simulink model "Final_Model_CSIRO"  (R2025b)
settings: Solver=ode23tb  StartTime=0.0  StopTime=50  RelTol=1e-3
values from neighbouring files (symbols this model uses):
  C_4 = 0.1670*C_b    (= 1.00487241952e-06)    [VSM_CSIRO.m]    (also in VSM.m)
  C_6 = 0.2835*C_b    (= 1.70587623314e-06)    [VSM_CSIRO.m]    (also in VSM.m)
  C_8 = 0.2275*C_b    (= 1.36891302659e-06)    [VSM_CSIRO.m]    (also in VSM.m)
  C_dc = 0.008*(n)    (= 1.6)    [VSM_CSIRO.m]    (also in VSM.m)
  C_f = n*300*10^-6    (= 0.06)    [VSM_CSIRO.m]    (also in VSM.m)
  D_p = (1/(m_p*w_b))    (= 101321.183642)    [VSM_CSIRO.m]    (also in VSM.m)
  droop_percentage = 1    [VSM_CSIRO.m]    (also in VSM.m = 5)
  i_ll = -1.15*(S_b/Vdc_n)-i_loss_dc    [VSM_CSIRO.m]    (also in VSM.m)
  i_ul = 1.15*(S_b/Vdc_n)+i_loss_dc    [VSM_CSIRO.m]    (also in VSM.m)
  J = D_p*tau_f    (= 2026.42367285)    [VSM_CSIRO.m]    (also in VSM.m)
  k_dc = eta_1/(Vdc_n*m_p)    [VSM_CSIRO.m]    (also in VSM.m)
  K_p = (1/Vdc_n)    [VSM_CSIRO.m]    (also in VSM.m)
  K_r = 1/R_dc    [VSM_CSIRO.m]    (also in VSM.m)
  Kff_i = 1    [VSM_CSIRO.m]    (also in VSM.m)
  Kff_v = 1    [VSM_CSIRO.m]    (also in VSM.m)
  Ki_i = (1/n)*1.19    (= 0.00595)    [VSM_CSIRO.m]    (also in VSM.m)
  Ki_v = (n)*1.161022    (= 232.2044)    [VSM_CSIRO.m]    (also in VSM.m)
  ki_v_ac = 4*5.2500e-04    (= 0.0021)    [VSM_CSIRO.m]    (also in VSM.m)
  Kp_i = 0.738891    [VSM_CSIRO.m]    (also in VSM.m)
  Kp_v = 0.52    [VSM_CSIRO.m]    (also in VSM.m)
  kp_v_ac = 0.001    [VSM_CSIRO.m]    (also in VSM.m)
  L1_pu = 1*0.0186/m    (= 0.000186)    [VSM_CSIRO.m]    (also in VSM.m)
  L_45 = L_lines(2)    [VSM_CSIRO.m]    (also in VSM.m)
  L_56 = L_lines(3)    [VSM_CSIRO.m]    (also in VSM.m)
  L_67 = L_lines(5)    [VSM_CSIRO.m]    (also in VSM.m)
  L_78 = L_lines(6)    [VSM_CSIRO.m]    (also in VSM.m)
  L_89 = L_lines(8)    [VSM_CSIRO.m]    (also in VSM.m)
  L_94 = L_lines(9)    [VSM_CSIRO.m]    (also in VSM.m)
  L_f = (1/n)*200*10^-6    (= 1e-06)    [VSM_CSIRO.m]    (also in VSM.m)
  n = 200    [VSM_CSIRO.m]    (also in VSM.m)
  pl = S_b*ps    (= 75000000)    [VSM_CSIRO.m]    (also in VSM.m)
  ps = base/3    (= 0.75)    [VSM_CSIRO.m]    (also in VSM.m)
  R1_pu = 1*0.00734/m    (= 7.34e-05)    [VSM_CSIRO.m]    (also in VSM.m)
  R_45 = R_lines(2)    [VSM_CSIRO.m]    (also in VSM.m)
  R_56 = R_lines(3)    [VSM_CSIRO.m]    (also in VSM.m)
  R_67 = R_lines(5)    [VSM_CSIRO.m]    (also in VSM.m)
  R_78 = R_lines(6)    [VSM_CSIRO.m]    (also in VSM.m)
  R_89 = R_lines(8)    [VSM_CSIRO.m]    (also in VSM.m)
  R_94 = R_lines(9)    [VSM_CSIRO.m]    (also in VSM.m)
  R_dc = (Vdc_n/(0.05*(S_b)/Vdc_n))    [VSM_CSIRO.m]    (also in VSM.m)
  R_f = 0.001/n    (= 5e-06)    [VSM_CSIRO.m]    (also in VSM.m)
  S_b = 100*(10^6)    (= 100000000)    [VSM_CSIRO.m]    (also in VSM.m)
  S_bt = S_b    (= 100000000)    [VSM_CSIRO.m]    (also in VSM.m)
  T_en = T_load-0.5    (= 44.5)    [VSM_CSIRO.m]    (also in VSM.m = 24.5)
  t_l = 2    [VSM_CSIRO.m]
  tau_dc = 0.05    [VSM_CSIRO.m]    (also in VSM.m)
  tau_g = 5    [VSM_CSIRO.m]    (also in VSM.m)
  V1_rms = 1000    [VSM_CSIRO.m]    (also in VSM.m)
  V2_rms = 13800    [VSM_CSIRO.m]    (also in VSM.m)
  V_m = sqrt(2/3)*V1_rms    [VSM_CSIRO.m]    (also in VSM.m)
  Vdc_n = 3*V_m    [VSM_CSIRO.m]    (also in VSM.m)
  w_b = 2*pi*f_b    (= 314.159265359)    [VSM_CSIRO.m]    (also in VSM.m)
  w_f = 2*pi*5    (= 31.4159265359)    [VSM_CSIRO.m]    (also in VSM.m)
undefined symbols (not defined in the file or in its folder): D1, Delta, DiscIntNeverNeededParam, i_dc
libraries: spsSeriesRLCBranchLib x142, spsThreePhaseVIMeasurementLib x69, slpidlib x44, spsabctodq0Lib x44, spsVoltageMeasurementLib x28, spsGroundLib x23, spsThreePhaseBreakerLib x23, spsThreePhaseParallelRLCLoadLib x21, spsdq0toabcLib x16, spsUniversalBridgeLib x16, spsPowerPositiveSequenceLib x14, spsDCVoltageSourceLib x14
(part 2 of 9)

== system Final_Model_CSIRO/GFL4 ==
  B1 : spsThreePhaseVIMeasurementLib/Three-Phase V-I Measurement  VoltageMeasurement=phase-to-ground  SetLabelV=on  LabelV=Vabc_B1_5  Vpu=off  VpuLL=off  CurrentMeasurement=yes  SetLabelI=on  LabelI=Iabc_B1_5  Ipu=off  Pbase=100e6  Vbase=500e3  OutputType=Complex  PhasorSimulation=off  PSBequivalent=0
  B3 : spsThreePhaseVIMeasurementLib/Three-Phase V-I Measurement  VoltageMeasurement=phase-to-ground  SetLabelV=on  LabelV=Vabc_B3_5  Vpu=off  VpuLL=off  CurrentMeasurement=yes  SetLabelI=on  LabelI=Iabc_B3_5  Ipu=off  Pbase=100e6  Vbase=500e3  OutputType=Complex  PhasorSimulation=off  PSBequivalent=0
  B4 : spsThreePhaseVIMeasurementLib/Three-Phase V-I Measurement  VoltageMeasurement=phase-to-ground  SetLabelV=on  LabelV=Vabc_B4_5  Vpu=off  VpuLL=off  CurrentMeasurement=yes  SetLabelI=on  LabelI=Iabc_B4_5  Ipu=off  Pbase=100e6  Vbase=500e3  OutputType=Complex  PhasorSimulation=off  PSBequivalent=0
  Constant1 : Constant  Value=0  SampleTime=-1
  Gain2 : Gain  Gain=1e-8
  Inverter Control : Subsystem
  LCL Filter : Subsystem
  Power (Positive-Sequence) : spsPowerPositiveSequenceLib/Power (Positive-Sequence)  Freq=50  Vinit=[0, 0]  Iinit=[0, 0]  Ts=0
  Scope : Scope  NumInputPorts=4
  Scope1 : Scope
  Step : Step  Time=12+3*t_l  After=8200  SampleTime=0
  Universal Bridge : spsUniversalBridgeLib/Universal Bridge  Arms=3  SnubberResistance=1e5  SnubberCapacitance=inf  Device=Average-model based VSC  Ron=1e-3  Lon=0  ForwardVoltages="[  0  0  ]"  ForwardVoltage=0  GTOparameters=[ 10e-6 , 20e-6 ]  IGBTparameters=[ 1e-6 , 2e-6 ]  Measurements=None  Measurements_2=None  converterType=Rectifier
  Vdc : spsDCVoltageSourceLib/DC Voltage Source  Amplitude=1800  Measurements=None
  Voltage Measurement1 : spsVoltageMeasurementLib/Voltage Measurement  PhasorSimulation=off  OutputType=Complex  PSBequivalent=0
  Connection Port : PMIOPort  Side=Left
  Connection Port1 : PMIOPort  Port=2  Side=Left
  Connection Port2 : PMIOPort  Port=3  Side=Left
  Out1 : Outport
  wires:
  [Vabc_B1_5] -> Scope/3  "Inverter Voltage"
  [Iabc_B1_5] -> Scope/4  "Inverter Current"
  Voltage Measurement1/1 -> Scope1/1
  [Iabc_B3_5] -> Power (Positive-Sequence)/2, Scope/2  "PCC Current"
  Inverter Control/1(Pulses) -> Universal Bridge/1
  [Vabc_B3_5] -> Inverter Control/1(Vabc_B3)
  [Iabc_B3_5] -> Inverter Control/2(Iabc_B3)
  [Vabc_B3_5] -> Scope/1, Power (Positive-Sequence)/1  "PCC Voltage"
  Power (Positive-Sequence)/1 -> Gain2/1
  Gain2/1 -> Out1/1
  Constant1/1 -> Inverter Control/4(Iqref)
  Step/1 -> Inverter Control/3(Idref)
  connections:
  Universal Bridge/RConn1 -- Vdc/RConn1
  Universal Bridge/RConn2 -- Vdc/LConn1
  B1/LConn2 -- Voltage Measurement1/LConn2 -- Universal Bridge/LConn2
  Universal Bridge/LConn1 -- Voltage Measurement1/LConn1 -- B1/LConn1
  B3/LConn3 -- LCL Filter/RConn3
  B3/RConn3 -- B4/LConn3
  B3/RConn1 -- B4/LConn1
  Connection Port2/RConn1 -- B4/RConn3
  B3/LConn2 -- LCL Filter/RConn2
  Universal Bridge/LConn3 -- B1/LConn3
  B3/RConn2 -- B4/LConn2
  B3/LConn1 -- LCL Filter/RConn1
  B1/RConn1 -- LCL Filter/LConn1
  B1/RConn2 -- LCL Filter/LConn2
  B1/RConn3 -- LCL Filter/LConn3
  B4/RConn1 -- Connection Port/RConn1
  B4/RConn2 -- Connection Port1/RConn1

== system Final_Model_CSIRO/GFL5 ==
  B1 : spsThreePhaseVIMeasurementLib/Three-Phase V-I Measurement  VoltageMeasurement=phase-to-ground  SetLabelV=on  LabelV=Vabc_B1_6  Vpu=off  VpuLL=off  CurrentMeasurement=yes  SetLabelI=on  LabelI=Iabc_B1_6  Ipu=off  Pbase=100e6  Vbase=500e3  OutputType=Complex  PhasorSimulation=off  PSBequivalent=0
  B3 : spsThreePhaseVIMeasurementLib/Three-Phase V-I Measurement  VoltageMeasurement=phase-to-ground  SetLabelV=on  LabelV=Vabc_B3_6  Vpu=off  VpuLL=off  CurrentMeasurement=yes  SetLabelI=on  LabelI=Iabc_B3_6  Ipu=off  Pbase=100e6  Vbase=500e3  OutputType=Complex  PhasorSimulation=off  PSBequivalent=0
  B4 : spsThreePhaseVIMeasurementLib/Three-Phase V-I Measurement  VoltageMeasurement=phase-to-ground  SetLabelV=on  LabelV=Vabc_B4_6  Vpu=off  VpuLL=off  CurrentMeasurement=yes  SetLabelI=on  LabelI=Iabc_B4_6  Ipu=off  Pbase=100e6  Vbase=500e3  OutputType=Complex  PhasorSimulation=off  PSBequivalent=0
  Constant1 : Constant  Value=0  SampleTime=-1
  Gain2 : Gain  Gain=1e-8
  Inverter Control : Subsystem
  LCL Filter : Subsystem
  Power (Positive-Sequence) : spsPowerPositiveSequenceLib/Power (Positive-Sequence)  Freq=50  Vinit=[0, 0]  Iinit=[0, 0]  Ts=0
  Scope : Scope  NumInputPorts=4
  Scope1 : Scope
  Step : Step  Time=12+4*t_l  After=8200  SampleTime=0
  Universal Bridge : spsUniversalBridgeLib/Universal Bridge  Arms=3  SnubberResistance=1e5  SnubberCapacitance=inf  Device=Average-model based VSC  Ron=1e-3  Lon=0  ForwardVoltages="[  0  0  ]"  ForwardVoltage=0  GTOparameters=[ 10e-6 , 20e-6 ]  IGBTparameters=[ 1e-6 , 2e-6 ]  Measurements=None  Measurements_2=None  converterType=Rectifier
  Vdc : spsDCVoltageSourceLib/DC Voltage Source  Amplitude=1800  Measurements=None
  Voltage Measurement1 : spsVoltageMeasurementLib/Voltage Measurement  PhasorSimulation=off  OutputType=Complex  PSBequivalent=0
  Connection Port : PMIOPort  Side=Left
  Connection Port1 : PMIOPort  Port=2  Side=Left
  Connection Port2 : PMIOPort  Port=3  Side=Left
  Out1 : Outport
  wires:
  [Vabc_B1_6] -> Scope/3  "Inverter Voltage"
  [Iabc_B1_6] -> Scope/4  "Inverter Current"
  Voltage Measurement1/1 -> Scope1/1
  [Iabc_B3_6] -> Power (Positive-Sequence)/2, Scope/2  "PCC Current"
  Inverter Control/1(Pulses) -> Universal Bridge/1
  [Vabc_B3_6] -> Inverter Control/1(Vabc_B3)
  [Iabc_B3_6] -> Inverter Control/2(Iabc_B3)
  [Vabc_B3_6] -> Scope/1, Power (Positive-Sequence)/1  "PCC Voltage"
  Power (Positive-Sequence)/1 -> Gain2/1
  Gain2/1 -> Out1/1
  Constant1/1 -> Inverter Control/4(Iqref)
  Step/1 -> Inverter Control/3(Idref)
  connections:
  Universal Bridge/RConn1 -- Vdc/RConn1
  Universal Bridge/RConn2 -- Vdc/LConn1
  B1/LConn2 -- Voltage Measurement1/LConn2 -- Universal Bridge/LConn2
  Universal Bridge/LConn1 -- Voltage Measurement1/LConn1 -- B1/LConn1
  B3/LConn3 -- LCL Filter/RConn3
  B3/RConn3 -- B4/LConn3
  B3/RConn1 -- B4/LConn1
  Connection Port2/RConn1 -- B4/RConn3
  B3/LConn2 -- LCL Filter/RConn2
  Universal Bridge/LConn3 -- B1/LConn3
  B3/RConn2 -- B4/LConn2
  B3/LConn1 -- LCL Filter/RConn1
  B1/RConn1 -- LCL Filter/LConn1
  B1/RConn2 -- LCL Filter/LConn2
  B1/RConn3 -- LCL Filter/LConn3
  B4/RConn1 -- Connection Port/RConn1
  B4/RConn2 -- Connection Port1/RConn1

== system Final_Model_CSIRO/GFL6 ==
  B1 : spsThreePhaseVIMeasurementLib/Three-Phase V-I Measurement  VoltageMeasurement=phase-to-ground  SetLabelV=on  LabelV=Vabc_B1_7  Vpu=off  VpuLL=off  CurrentMeasurement=yes  SetLabelI=on  LabelI=Iabc_B1_7  Ipu=off  Pbase=100e6  Vbase=500e3  OutputType=Complex  PhasorSimulation=off  PSBequivalent=0
  B3 : spsThreePhaseVIMeasurementLib/Three-Phase V-I Measurement  VoltageMeasurement=phase-to-ground  SetLabelV=on  LabelV=Vabc_B3_7  Vpu=off  VpuLL=off  CurrentMeasurement=yes  SetLabelI=on  LabelI=Iabc_B3_7  Ipu=off  Pbase=100e6  Vbase=500e3  OutputType=Complex  PhasorSimulation=off  PSBequivalent=0
  B4 : spsThreePhaseVIMeasurementLib/Three-Phase V-I Measurement  VoltageMeasurement=phase-to-ground  SetLabelV=on  LabelV=Vabc_B4_7  Vpu=off  VpuLL=off  CurrentMeasurement=yes  SetLabelI=on  LabelI=Iabc_B4_7  Ipu=off  Pbase=100e6  Vbase=500e3  OutputType=Complex  PhasorSimulation=off  PSBequivalent=0
  Constant1 : Constant  Value=0  SampleTime=-1
  Gain2 : Gain  Gain=1e-8
  Inverter Control : Subsystem
  LCL Filter : Subsystem
  Power (Positive-Sequence) : spsPowerPositiveSequenceLib/Power (Positive-Sequence)  Freq=50  Vinit=[0, 0]  Iinit=[0, 0]  Ts=0
  Scope : Scope  NumInputPorts=4
  Scope1 : Scope
  Step : Step  Time=12+5*t_l  After=8200  SampleTime=0
  Universal Bridge : spsUniversalBridgeLib/Universal Bridge  Arms=3  SnubberResistance=1e5  SnubberCapacitance=inf  Device=Average-model based VSC  Ron=1e-3  Lon=0  ForwardVoltages="[  0  0  ]"  ForwardVoltage=0  GTOparameters=[ 10e-6 , 20e-6 ]  IGBTparameters=[ 1e-6 , 2e-6 ]  Measurements=None  Measurements_2=None  converterType=Rectifier
  Vdc : spsDCVoltageSourceLib/DC Voltage Source  Amplitude=1800  Measurements=None
  Voltage Measurement1 : spsVoltageMeasurementLib/Voltage Measurement  PhasorSimulation=off  OutputType=Complex  PSBequivalent=0
  Connection Port : PMIOPort  Side=Left
  Connection Port1 : PMIOPort  Port=2  Side=Left
  Connection Port2 : PMIOPort  Port=3  Side=Left
  Out1 : Outport
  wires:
  [Vabc_B1_7] -> Scope/3  "Inverter Voltage"
  [Iabc_B1_7] -> Scope/4  "Inverter Current"
  Voltage Measurement1/1 -> Scope1/1
  [Iabc_B3_7] -> Power (Positive-Sequence)/2, Scope/2  "PCC Current"
  Inverter Control/1(Pulses) -> Universal Bridge/1
  [Vabc_B3_7] -> Inverter Control/1(Vabc_B3)
  [Iabc_B3_7] -> Inverter Control/2(Iabc_B3)
  [Vabc_B3_7] -> Scope/1, Power (Positive-Sequence)/1  "PCC Voltage"
  Power (Positive-Sequence)/1 -> Gain2/1
  Gain2/1 -> Out1/1
  Constant1/1 -> Inverter Control/4(Iqref)
  Step/1 -> Inverter Control/3(Idref)
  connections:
  Universal Bridge/RConn1 -- Vdc/RConn1
  Universal Bridge/RConn2 -- Vdc/LConn1
  B1/LConn2 -- Voltage Measurement1/LConn2 -- Universal Bridge/LConn2
  Universal Bridge/LConn1 -- Voltage Measurement1/LConn1 -- B1/LConn1
  B3/LConn3 -- LCL Filter/RConn3
  B3/RConn3 -- B4/LConn3
  B3/RConn1 -- B4/LConn1
  Connection Port2/RConn1 -- B4/RConn3
  B3/LConn2 -- LCL Filter/RConn2
  Universal Bridge/LConn3 -- B1/LConn3
  B3/RConn2 -- B4/LConn2
  B3/LConn1 -- LCL Filter/RConn1
  B1/RConn1 -- LCL Filter/LConn1
  B1/RConn2 -- LCL Filter/LConn2
  B1/RConn3 -- LCL Filter/LConn3
  B4/RConn1 -- Connection Port/RConn1
  B4/RConn2 -- Connection Port1/RConn1

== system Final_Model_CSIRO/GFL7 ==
  B1 : spsThreePhaseVIMeasurementLib/Three-Phase V-I Measurement  VoltageMeasurement=phase-to-ground  SetLabelV=on  LabelV=Vabc_B1_8  Vpu=off  VpuLL=off  CurrentMeasurement=yes  SetLabelI=on  LabelI=Iabc_B1_8  Ipu=off  Pbase=100e6  Vbase=500e3  OutputType=Complex  PhasorSimulation=off  PSBequivalent=0
  B3 : spsThreePhaseVIMeasurementLib/Three-Phase V-I Measurement  VoltageMeasurement=phase-to-ground  SetLabelV=on  LabelV=Vabc_B3_8  Vpu=off  VpuLL=off  CurrentMeasurement=yes  SetLabelI=on  LabelI=Iabc_B3_8  Ipu=off  Pbase=100e6  Vbase=500e3  OutputType=Complex  PhasorSimulation=off  PSBequivalent=0
  B4 : spsThreePhaseVIMeasurementLib/Three-Phase V-I Measurement  VoltageMeasurement=phase-to-ground  SetLabelV=on  LabelV=Vabc_B4_8  Vpu=off  VpuLL=off  CurrentMeasurement=yes  SetLabelI=on  LabelI=Iabc_B4_8  Ipu=off  Pbase=100e6  Vbase=500e3  OutputType=Complex  PhasorSimulation=off  PSBequivalent=0
  Constant1 : Constant  Value=0  SampleTime=-1
  Gain2 : Gain  Gain=1e-8
  Inverter Control : Subsystem
  LCL Filter : Subsystem
  Power (Positive-Sequence) : spsPowerPositiveSequenceLib/Power (Positive-Sequence)  Freq=50  Vinit=[0, 0]  Iinit=[0, 0]  Ts=0
  Scope : Scope  NumInputPorts=4
  Scope1 : Scope
  Step : Step  Time=12+6*t_l  After=8200  SampleTime=0
  Universal Bridge : spsUniversalBridgeLib/Universal Bridge  Arms=3  SnubberResistance=1e5  SnubberCapacitance=inf  Device=Average-model based VSC  Ron=1e-3  Lon=0  ForwardVoltages="[  0  0  ]"  ForwardVoltage=0  GTOparameters=[ 10e-6 , 20e-6 ]  IGBTparameters=[ 1e-6 , 2e-6 ]  Measurements=None  Measurements_2=None  converterType=Rectifier
  Vdc : spsDCVoltageSourceLib/DC Voltage Source  Amplitude=1800  Measurements=None
  Voltage Measurement1 : spsVoltageMeasurementLib/Voltage Measurement  PhasorSimulation=off  OutputType=Complex  PSBequivalent=0
  Connection Port : PMIOPort  Side=Left
  Connection Port1 : PMIOPort  Port=2  Side=Left
  Connection Port2 : PMIOPort  Port=3  Side=Left
  Out1 : Outport
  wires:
  [Vabc_B1_8] -> Scope/3  "Inverter Voltage"
  [Iabc_B1_8] -> Scope/4  "Inverter Current"
  Voltage Measurement1/1 -> Scope1/1
  [Iabc_B3_8] -> Power (Positive-Sequence)/2, Scope/2  "PCC Current"
  Inverter Control/1(Pulses) -> Universal Bridge/1
  [Vabc_B3_8] -> Inverter Control/1(Vabc_B3)
  [Iabc_B3_8] -> Inverter Control/2(Iabc_B3)
  [Vabc_B3_8] -> Scope/1, Power (Positive-Sequence)/1  "PCC Voltage"
  Power (Positive-Sequence)/1 -> Gain2/1
  Gain2/1 -> Out1/1
  Constant1/1 -> Inverter Control/4(Iqref)
  Step/1 -> Inverter Control/3(Idref)
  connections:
  Universal Bridge/RConn1 -- Vdc/RConn1
  Universal Bridge/RConn2 -- Vdc/LConn1
  B1/LConn2 -- Voltage Measurement1/LConn2 -- Universal Bridge/LConn2
  Universal Bridge/LConn1 -- Voltage Measurement1/LConn1 -- B1/LConn1
  B3/LConn3 -- LCL Filter/RConn3
  B3/RConn3 -- B4/LConn3
  B3/RConn1 -- B4/LConn1
  Connection Port2/RConn1 -- B4/RConn3
  B3/LConn2 -- LCL Filter/RConn2
  Universal Bridge/LConn3 -- B1/LConn3
  B3/RConn2 -- B4/LConn2
  B3/LConn1 -- LCL Filter/RConn1
  B1/RConn1 -- LCL Filter/LConn1
  B1/RConn2 -- LCL Filter/LConn2
  B1/RConn3 -- LCL Filter/LConn3
  B4/RConn1 -- Connection Port/RConn1
  B4/RConn2 -- Connection Port1/RConn1

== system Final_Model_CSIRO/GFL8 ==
  B1 : spsThreePhaseVIMeasurementLib/Three-Phase V-I Measurement  VoltageMeasurement=phase-to-ground  SetLabelV=on  LabelV=Vabc_B1_9  Vpu=off  VpuLL=off  CurrentMeasurement=yes  SetLabelI=on  LabelI=Iabc_B1_9  Ipu=off  Pbase=100e6  Vbase=500e3  OutputType=Complex  PhasorSimulation=off  PSBequivalent=0
  B3 : spsThreePhaseVIMeasurementLib/Three-Phase V-I Measurement  VoltageMeasurement=phase-to-ground  SetLabelV=on  LabelV=Vabc_B3_9  Vpu=off  VpuLL=off  CurrentMeasurement=yes  SetLabelI=on  LabelI=Iabc_B3_9  Ipu=off  Pbase=100e6  Vbase=500e3  OutputType=Complex  PhasorSimulation=off  PSBequivalent=0
  B4 : spsThreePhaseVIMeasurementLib/Three-Phase V-I Measurement  VoltageMeasurement=phase-to-ground  SetLabelV=on  LabelV=Vabc_B4_9  Vpu=off  VpuLL=off  CurrentMeasurement=yes  SetLabelI=on  LabelI=Iabc_B4_9  Ipu=off  Pbase=100e6  Vbase=500e3  OutputType=Complex  PhasorSimulation=off  PSBequivalent=0
  Constant1 : Constant  Value=0  SampleTime=-1
  Gain2 : Gain  Gain=1e-8
  Inverter Control : Subsystem
  LCL Filter : Subsystem
  Power (Positive-Sequence) : spsPowerPositiveSequenceLib/Power (Positive-Sequence)  Freq=50  Vinit=[0, 0]  Iinit=[0, 0]  Ts=0
  Scope : Scope  NumInputPorts=4
  Scope1 : Scope
  Step : Step  Time=12+7*t_l  After=8200  SampleTime=0
  Universal Bridge : spsUniversalBridgeLib/Universal Bridge  Arms=3  SnubberResistance=1e5  SnubberCapacitance=inf  Device=Average-model based VSC  Ron=1e-3  Lon=0  ForwardVoltages="[  0  0  ]"  ForwardVoltage=0  GTOparameters=[ 10e-6 , 20e-6 ]  IGBTparameters=[ 1e-6 , 2e-6 ]  Measurements=None  Measurements_2=None  converterType=Rectifier
  Vdc : spsDCVoltageSourceLib/DC Voltage Source  Amplitude=1800  Measurements=None
  Voltage Measurement1 : spsVoltageMeasurementLib/Voltage Measurement  PhasorSimulation=off  OutputType=Complex  PSBequivalent=0
  Connection Port : PMIOPort  Side=Left
  Connection Port1 : PMIOPort  Port=2  Side=Left
  Connection Port2 : PMIOPort  Port=3  Side=Left
  Out1 : Outport
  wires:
  [Vabc_B1_9] -> Scope/3  "Inverter Voltage"
  [Iabc_B1_9] -> Scope/4  "Inverter Current"
  Voltage Measurement1/1 -> Scope1/1
  [Iabc_B3_9] -> Power (Positive-Sequence)/2, Scope/2  "PCC Current"
  Inverter Control/1(Pulses) -> Universal Bridge/1
  [Vabc_B3_9] -> Inverter Control/1(Vabc_B3)
  [Iabc_B3_9] -> Inverter Control/2(Iabc_B3)
  [Vabc_B3_9] -> Scope/1, Power (Positive-Sequence)/1  "PCC Voltage"
  Power (Positive-Sequence)/1 -> Gain2/1
  Gain2/1 -> Out1/1
  Constant1/1 -> Inverter Control/4(Iqref)
  Step/1 -> Inverter Control/3(Idref)
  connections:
  Universal Bridge/RConn1 -- Vdc/RConn1
  Universal Bridge/RConn2 -- Vdc/LConn1
  B1/LConn2 -- Voltage Measurement1/LConn2 -- Universal Bridge/LConn2
  Universal Bridge/LConn1 -- Voltage Measurement1/LConn1 -- B1/LConn1
  B3/LConn3 -- LCL Filter/RConn3
  B3/RConn3 -- B4/LConn3
  B3/RConn1 -- B4/LConn1
  Connection Port2/RConn1 -- B4/RConn3
  B3/LConn2 -- LCL Filter/RConn2
  Universal Bridge/LConn3 -- B1/LConn3
  B3/RConn2 -- B4/LConn2
  B3/LConn1 -- LCL Filter/RConn1
  B1/RConn1 -- LCL Filter/LConn1
  B1/RConn2 -- LCL Filter/LConn2
  B1/RConn3 -- LCL Filter/LConn3
  B4/RConn1 -- Connection Port/RConn1
  B4/RConn2 -- Connection Port1/RConn1

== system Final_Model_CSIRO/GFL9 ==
  B1 : spsThreePhaseVIMeasurementLib/Three-Phase V-I Measurement  VoltageMeasurement=phase-to-ground  SetLabelV=on  LabelV=Vabc_B1_11  Vpu=off  VpuLL=off  CurrentMeasurement=yes  SetLabelI=on  LabelI=Iabc_B1_11  Ipu=off  Pbase=100e6  Vbase=500e3  OutputType=Complex  PhasorSimulation=off  PSBequivalent=0
  B3 : spsThreePhaseVIMeasurementLib/Three-Phase V-I Measurement  VoltageMeasurement=phase-to-ground  SetLabelV=on  LabelV=Vabc_B3_11  Vpu=off  VpuLL=off  CurrentMeasurement=yes  SetLabelI=on  LabelI=Iabc_B3_11  Ipu=off  Pbase=100e6  Vbase=500e3  OutputType=Complex  PhasorSimulation=off  PSBequivalent=0
  B4 : spsThreePhaseVIMeasurementLib/Three-Phase V-I Measurement  VoltageMeasurement=phase-to-ground  SetLabelV=on  LabelV=Vabc_B4_11  Vpu=off  VpuLL=off  CurrentMeasurement=yes  SetLabelI=on  LabelI=Iabc_B4_11  Ipu=off  Pbase=100e6  Vbase=500e3  OutputType=Complex  PhasorSimulation=off  PSBequivalent=0
  Constant1 : Constant  Value=0  SampleTime=-1
  Gain2 : Gain  Gain=1e-8
  Inverter Control : Subsystem
  LCL Filter : Subsystem
  Power (Positive-Sequence) : spsPowerPositiveSequenceLib/Power (Positive-Sequence)  Freq=50  Vinit=[0, 0]  Iinit=[0, 0]  Ts=0
  Scope : Scope  NumInputPorts=4
  Scope1 : Scope
  Step : Step  Time=12+8*t_l  After=8200  SampleTime=0
  Universal Bridge : spsUniversalBridgeLib/Universal Bridge  Arms=3  SnubberResistance=1e5  SnubberCapacitance=inf  Device=Average-model based VSC  Ron=1e-3  Lon=0  ForwardVoltages="[  0  0  ]"  ForwardVoltage=0  GTOparameters=[ 10e-6 , 20e-6 ]  IGBTparameters=[ 1e-6 , 2e-6 ]  Measurements=None  Measurements_2=None  converterType=Rectifier
  Vdc : spsDCVoltageSourceLib/DC Voltage Source  Amplitude=1800  Measurements=None
  Voltage Measurement1 : spsVoltageMeasurementLib/Voltage Measurement  PhasorSimulation=off  OutputType=Complex  PSBequivalent=0
  Connection Port : PMIOPort  Side=Left
  Connection Port1 : PMIOPort  Port=2  Side=Left
  Connection Port2 : PMIOPort  Port=3  Side=Left
  Out1 : Outport
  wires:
  [Vabc_B1_11] -> Scope/3  "Inverter Voltage"
  [Iabc_B1_11] -> Scope/4  "Inverter Current"
  Voltage Measurement1/1 -> Scope1/1
  [Iabc_B3_11] -> Power (Positive-Sequence)/2, Scope/2  "PCC Current"
  Inverter Control/1(Pulses) -> Universal Bridge/1
  [Vabc_B3_11] -> Inverter Control/1(Vabc_B3)
  [Iabc_B3_11] -> Inverter Control/2(Iabc_B3)
  [Vabc_B3_11] -> Scope/1, Power (Positive-Sequence)/1  "PCC Voltage"
  Power (Positive-Sequence)/1 -> Gain2/1
  Gain2/1 -> Out1/1
  Constant1/1 -> Inverter Control/4(Iqref)
  Step/1 -> Inverter Control/3(Idref)
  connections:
  Universal Bridge/RConn1 -- Vdc/RConn1
  Universal Bridge/RConn2 -- Vdc/LConn1
  B1/LConn2 -- Voltage Measurement1/LConn2 -- Universal Bridge/LConn2
  Universal Bridge/LConn1 -- Voltage Measurement1/LConn1 -- B1/LConn1
  B3/LConn3 -- LCL Filter/RConn3
  B3/RConn3 -- B4/LConn3
  B3/RConn1 -- B4/LConn1
  Connection Port2/RConn1 -- B4/RConn3
  B3/LConn2 -- LCL Filter/RConn2
  Universal Bridge/LConn3 -- B1/LConn3
  B3/RConn2 -- B4/LConn2
  B3/LConn1 -- LCL Filter/RConn1
  B1/RConn1 -- LCL Filter/LConn1
  B1/RConn2 -- LCL Filter/LConn2
  B1/RConn3 -- LCL Filter/LConn3
  B4/RConn1 -- Connection Port/RConn1
  B4/RConn2 -- Connection Port1/RConn1

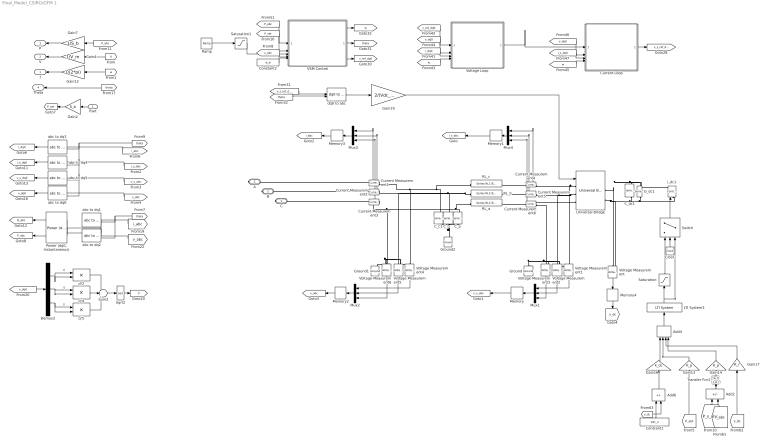
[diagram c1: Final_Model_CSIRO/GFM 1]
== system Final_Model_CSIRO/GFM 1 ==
  Pset : Inport
  Add2 : Sum  Inputs=+-
  Add4 : Sum  Inputs=++++
  Add6 : Sum  Inputs=+-
  C_a : spsSeriesRLCBranchLib/Series RLC Branch  LConnTagsString=__new0  RConnTagsString=__new0  BranchType=C  Resistance=1  Inductance=1e-3  SetiL0=off  InitialCurrent=0  Capacitance=C_f  Setx0=off  InitialVoltage=165  Measurements=None
  C_b : spsSeriesRLCBranchLib/Series RLC Branch  LConnTagsString=__new0  RConnTagsString=__new0  BranchType=C  Resistance=1  Inductance=1e-3  SetiL0=off  InitialCurrent=0  Capacitance=C_f  Setx0=off  InitialVoltage=165  Measurements=None
  C_c1 : spsSeriesRLCBranchLib/Series RLC Branch  LConnTagsString=__new0  RConnTagsString=__new0  BranchType=C  Resistance=1  Inductance=1e-3  SetiL0=off  InitialCurrent=0  Capacitance=C_f  Setx0=off  InitialVoltage=165  Measurements=None
  C_dc1 : spsSeriesRLCBranchLib/Series RLC Branch  LConnTagsString=__new0  RConnTagsString=__new0  BranchType=C  Resistance=1  Inductance=1e-3  SetiL0=off  InitialCurrent=0  Capacitance=C_dc  Setx0=off  InitialVoltage=Vdc_n  Measurements=None
  Clock : Clock
  Constant1 : Constant  Value=Vdc_n
  Constant2 : Constant  Value=w_b
  Current Loop : Subsystem
  Current Measurement{1..6} (6 alike) : spsCurrentMeasurementLib/Current Measurement  PhasorSimulation=off  OutputType=Complex  PSBequivalent=0
  Demux2 : Demux  Outputs=3
  G_dc1 : spsSeriesRLCBranchLib/Series RLC Branch  LConnTagsString=__new0  RConnTagsString=__new0  BranchType=R  Resistance=R_dc  Inductance=1e-3  SetiL0=off  InitialCurrent=0  Capacitance=1e-6  Setx0=off  InitialVoltage=0  Measurements=None
  Gain12 : Gain  Gain=1/(2*pi)
  Gain13 : Gain  Gain=K_p
  Gain14 : Gain  Gain=K_p
  Gain16 : Gain  Gain=k_dc
  Gain17 : Gain  Gain=K_r
  Gain19 : Gain  Gain=2/(Vdc_n)
  Gain2 : Gain  Gain=S_b
  Gain4 : Gain  Gain=1/V_m
  Gain7 : Gain  Gain=1/S_b
  Ground : spsGroundLib/Ground  LConnTagsString=a
  Ground1 : spsGroundLib/Ground  LConnTagsString=a
  Ground2 : spsGroundLib/Ground  LConnTagsString=a
  LTI System3 : cstblocks/LTI System  sys=tf(1,[tau_dc 1])  IC=[]  PadeOrder=0
  Memory{,1..4} (5 alike) : Memory
  Mux{1..4} (4 alike) : Mux  Inputs=3
  "Power (dq0, Instantaneous)" : spsPowerdq0InstantaneousLib/Power (dq0, Instantaneous)
  RL_a : spsSeriesRLCBranchLib/Series RLC Branch  LConnTagsString=__new0  RConnTagsString=__new0  BranchType=RL  Resistance=R_f  Inductance=L_f  SetiL0=off  InitialCurrent=0  Capacitance=1e-6  Setx0=off  InitialVoltage=0  Measurements=Branch voltage and current
  RL_b : spsSeriesRLCBranchLib/Series RLC Branch  LConnTagsString=__new0  RConnTagsString=__new0  BranchType=RL  Resistance=R_f  Inductance=L_f  SetiL0=off  InitialCurrent=0  Capacitance=1e-6  Setx0=off  InitialVoltage=0  Measurements=None
  RL_c : spsSeriesRLCBranchLib/Series RLC Branch  LConnTagsString=__new0  RConnTagsString=__new0  BranchType=RL  Resistance=R_f  Inductance=L_f  SetiL0=off  InitialCurrent=0  Capacitance=1e-6  Setx0=off  InitialVoltage=0  Measurements=None
  Ramp : simulink/Sources/Ramp  slope=500  start=0  InitialOutput=0
  Saturation : Saturate  UpperLimit=i_ul  LowerLimit=i_ll
  Saturation1 : Saturate  UpperLimit=V_m  LowerLimit=0
  Sqrt2 : Sqrt
  Sum2 : Sum  Inputs=+++  InputSameDT=on  SaturateOnIntegerOverflow=on
  Switch : Switch  Criteria=u2 > Threshold  Threshold=T_en
  Transfer Fcn2 : TransferFcn  Numerator=[w_f]  Denominator=[1 w_f]
  Universal Bridge : spsUniversalBridgeLib/Universal Bridge  Arms=3  SnubberResistance=1e5  SnubberCapacitance=inf  Device=Average-model based VSC  Ron=1e-3  Lon=0  ForwardVoltages="[  0  0  ]"  ForwardVoltage=0  GTOparameters=[ 10e-6 , 20e-6 ]  IGBTparameters=[ 1e-6 , 2e-6 ]  Measurements=None  Measurements_2=None  converterType=Rectifier
  VSM Control : Subsystem
  Voltage Loop : Subsystem
  Voltage Measurement{,1..6} (7 alike) : spsVoltageMeasurementLib/Voltage Measurement  PhasorSimulation=off  OutputType=Complex  PSBequivalent=0
  abc to dq{1..6} (6 alike) : spsabctodq0Lib/abc to dq0  Alignment=90 degrees behind phase A axis
  dq0 to abc : spsdq0toabcLib/dq0 to abc  Alignment=90 degrees behind phase A axis
  d²2 : Product  InputSameDT=on  RndMeth=Zero  SaturateOnIntegerOverflow=on
  i_dc1 : spsControlledCurrentSourceLib/Controlled Current Source  Initialize=off  Source_Type=DC  Amplitude=i_dc  Phase=0  Frequency=0  Measurements=None
  q²4 : Product  InputSameDT=on  RndMeth=Zero  SaturateOnIntegerOverflow=on
  q²5 : Product  InputSameDT=on  RndMeth=Zero  SaturateOnIntegerOverflow=on
  C : PMIOPort  Side=Right
  B : PMIOPort  Port=2  Side=Right
  A : PMIOPort  Port=3  Side=Right
  f : Outport  VectorParamsAs1DForOutWhenUnconnected=off
  V : Outport  Port=2  VectorParamsAs1DForOutWhenUnconnected=off
  P : Outport  Port=3  VectorParamsAs1DForOutWhenUnconnected=off
  Theta : Outport  Port=4  VectorParamsAs1DForOutWhenUnconnected=off
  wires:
  Add4/1 -> LTI System3/1
  Clock/1 -> Switch/2
  Saturation/1 -> Switch/1
  LTI System3/1 -> Switch/3, Saturation/1
  Gain7/1 -> P/1
  [P_abc] -> Gain7/1
  Current Measurement6/1 -> Mux4/3
  Current Measurement5/1 -> Mux4/2
  Current Measurement4/1 -> Mux4/1
  Current Measurement3/1 -> Mux3/3
  Current Measurement2/1 -> Mux3/2
  Current Measurement1/1 -> Mux3/1
  Voltage Measurement4/1 -> Mux2/1
  Voltage Measurement5/1 -> Mux2/2
  Voltage Measurement6/1 -> Mux2/3
  Voltage Measurement3/1 -> Mux1/3
  Voltage Measurement2/1 -> Mux1/2
  Voltage Measurement1/1 -> Mux1/1
  [V] -> Gain4/1
  Gain2/1 -> [P_set]
  Pset/1 -> Gain2/1
  Gain12/1 -> f/1
  [w] -> Gain12/1
  Mux2/1 -> Memory2/1
  Mux3/1 -> Memory3/1
  Mux1/1 -> Memory/1
  abc to dq1/1 -> "Power (dq0, Instantaneous)"/2
  abc to dq2/1 -> "Power (dq0, Instantaneous)"/1
  [theta] -> abc to dq2/2, abc to dq1/2
  [v_abc] -> abc to dq2/1
  "Power (dq0, Instantaneous)"/2 -> [Q_abc]
  "Power (dq0, Instantaneous)"/1 -> [P_abc]
  [i_abc] -> abc to dq1/1
  Gain4/1 -> V/1
  [theta] -> Theta/1
  [i_abc] -> abc to dq3/1
  [i_s_abc] -> abc to dq4/1
  [v_abc] -> abc to dq6/1
  [v_s_abc] -> abc to dq5/1
  [theta] -> abc to dq4/2, abc to dq5/2, abc to dq6/2, abc to dq3/2
  abc to dq3/1 -> [i_dq0]
  abc to dq4/1 -> [i_s_dq0]
  abc to dq5/1 -> [v_s_dq0]
  abc to dq6/1 -> [v_dq0]
  [theta] -> dq0 to abc/2
  q²4/1 -> Sum2/2
  [v_dq0] -> Demux2/1
  q²5/1 -> Sum2/3
  Sum2/1 -> Sqrt2/1
  Demux2/3 -> q²5/1, q²5/2  "0"
  d²2/1 -> Sum2/1
  Demux2/2 -> q²4/1, q²4/2  "q"
  Demux2/1 -> d²2/1, d²2/2  "d"
  Sqrt2/1 -> [V]
  Mux4/1 -> Memory1/1
  Memory2/1 -> [v_abc]
  Memory3/1 -> [i_abc]
  Voltage Measurement/1 -> Memory4/1
  Memory4/1 -> [v_dc]
  Memory/1 -> [v_s_abc]
  Memory1/1 -> [i_s_abc]
  dq0 to abc/1 -> Gain19/1
  [w] -> Current Loop/4(w)
  [v_ref_dq0] -> Voltage Loop/1(v_ref_dq0)
  [i_dq0] -> Voltage Loop/3(i_dq0)
  Voltage Loop/1(i_s_ref_dq0) -> Current Loop/1(i_s_ref_dq0)
  [v_dq0] -> Current Loop/2(v_dq0)
  [i_s_dq0] -> Current Loop/3(i_s_dq0)
  Current Loop/1(v_s_ref_dq0) -> [v_s_ref_dq0]
  [w] -> Voltage Loop/4(w)
  [v_dq0] -> Voltage Loop/2(v_dq0)
  Switch/1 -> i_dc1/1
  Gain19/1 -> Universal Bridge/1
  [v_s_ref_dq0] -> dq0 to abc/1
  VSM Control/2(theta_ref) -> [theta]
  VSM Control/3(v_ref_dq0) -> [v_ref_dq0]
  Constant2/1 -> VSM Control/5(w_b)
  [P_set] -> VSM Control/2(p_set)
  [v_abc] -> VSM Control/4(V_abc)
  [P_abc] -> VSM Control/1(p_m)
  VSM Control/1(w_ref) -> [w]
  [P_abc] -> Add2/2
  Gain14/1 -> Add4/4
  [P_set] -> Gain13/1
  Gain13/1 -> Add4/2
  Gain16/1 -> Add4/1
  Constant1/1 -> Add6/1
  Gain17/1 -> Add4/3
  Add2/1 -> Transfer Fcn2/1
  Transfer Fcn2/1 -> Gain14/1
  [v_dc] -> Add6/2
  Add6/1 -> Gain16/1
  [P_s_abc] -> Add2/1
  [v_dc] -> Gain17/1
  Ramp/1 -> Saturation1/1
  Saturation1/1 -> VSM Control/3(v_m)
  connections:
  RL_b/RConn1 -- Voltage Measurement5/LConn1 -- Current Measurement2/LConn1 -- C_b/LConn1
  Voltage Measurement6/LConn1 -- Current Measurement3/LConn1 -- C_a/LConn1 -- RL_a/RConn1
  Current Measurement4/RConn1 -- RL_c/LConn1
  Current Measurement6/RConn1 -- RL_a/LConn1
  Current Measurement5/RConn1 -- RL_b/LConn1
  Voltage Measurement/LConn1 -- Universal Bridge/RConn1 -- C_dc1/LConn1 -- G_dc1/LConn1 -- i_dc1/RConn1
  Voltage Measurement6/LConn2 -- Voltage Measurement5/LConn2 -- Voltage Measurement4/LConn2 -- Ground1/LConn1
  Ground/LConn1 -- Voltage Measurement2/LConn2 -- Voltage Measurement1/LConn2 -- Voltage Measurement3/LConn2
  Current Measurement3/RConn1 -- C/RConn1
  Current Measurement2/RConn1 -- B/RConn1
  Current Measurement1/RConn1 -- A/RConn1
  Current Measurement6/LConn1 -- Universal Bridge/LConn3 -- Voltage Measurement3/LConn1
  Universal Bridge/LConn2 -- Current Measurement5/LConn1 -- Voltage Measurement2/LConn1
  Universal Bridge/LConn1 -- Current Measurement4/LConn1 -- Voltage Measurement1/LConn1
  Universal Bridge/RConn2 -- Voltage Measurement/LConn2 -- C_dc1/RConn1 -- G_dc1/RConn1 -- i_dc1/LConn1
  C_b/RConn1 -- C_a/RConn1 -- Ground2/LConn1 -- C_c1/RConn1
  Voltage Measurement4/LConn1 -- Current Measurement1/LConn1 -- C_c1/LConn1 -- RL_c/RConn1

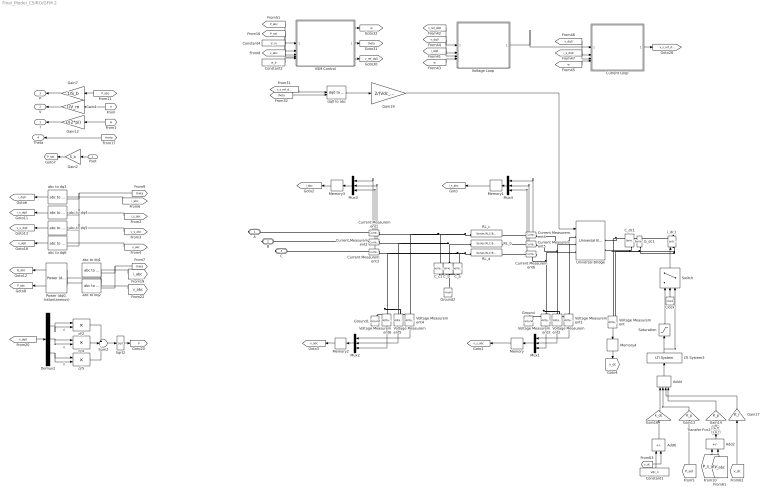
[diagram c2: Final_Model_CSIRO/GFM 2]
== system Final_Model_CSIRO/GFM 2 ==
  Pset : Inport
  Add2 : Sum  Inputs=+-
  Add4 : Sum  Inputs=++++
  Add6 : Sum  Inputs=+-
  C_a : spsSeriesRLCBranchLib/Series RLC Branch  LConnTagsString=__new0  RConnTagsString=__new0  BranchType=C  Resistance=1  Inductance=1e-3  SetiL0=off  InitialCurrent=0  Capacitance=C_f  Setx0=off  InitialVoltage=165  Measurements=None
  C_b : spsSeriesRLCBranchLib/Series RLC Branch  LConnTagsString=__new0  RConnTagsString=__new0  BranchType=C  Resistance=1  Inductance=1e-3  SetiL0=off  InitialCurrent=0  Capacitance=C_f  Setx0=off  InitialVoltage=165  Measurements=None
  C_c1 : spsSeriesRLCBranchLib/Series RLC Branch  LConnTagsString=__new0  RConnTagsString=__new0  BranchType=C  Resistance=1  Inductance=1e-3  SetiL0=off  InitialCurrent=0  Capacitance=C_f  Setx0=off  InitialVoltage=165  Measurements=None
  C_dc1 : spsSeriesRLCBranchLib/Series RLC Branch  LConnTagsString=__new0  RConnTagsString=__new0  BranchType=C  Resistance=1  Inductance=1e-3  SetiL0=off  InitialCurrent=0  Capacitance=C_dc  Setx0=off  InitialVoltage=Vdc_n  Measurements=None
  Clock : Clock
  Constant1 : Constant  Value=Vdc_n
  Constant2 : Constant  Value=w_b
  Constant4 : Constant  Value=V_m
  Current Loop : Subsystem
  Current Measurement{1..6} (6 alike) : spsCurrentMeasurementLib/Current Measurement  PhasorSimulation=off  OutputType=Complex  PSBequivalent=0
  Demux2 : Demux  Outputs=3
  G_dc1 : spsSeriesRLCBranchLib/Series RLC Branch  LConnTagsString=__new0  RConnTagsString=__new0  BranchType=R  Resistance=R_dc  Inductance=1e-3  SetiL0=off  InitialCurrent=0  Capacitance=1e-6  Setx0=off  InitialVoltage=0  Measurements=None
  Gain12 : Gain  Gain=1/(2*pi)
  Gain13 : Gain  Gain=K_p
  Gain14 : Gain  Gain=K_p
  Gain16 : Gain  Gain=k_dc
  Gain17 : Gain  Gain=K_r
  Gain19 : Gain  Gain=2/(Vdc_n)
  Gain2 : Gain  Gain=S_b
  Gain4 : Gain  Gain=1/V_m
  Gain7 : Gain  Gain=1/S_b
  Ground : spsGroundLib/Ground  LConnTagsString=a
  Ground1 : spsGroundLib/Ground  LConnTagsString=a
  Ground2 : spsGroundLib/Ground  LConnTagsString=a
  LTI System3 : cstblocks/LTI System  sys=tf(1,[tau_dc 1])  IC=[]  PadeOrder=0
  Memory{,1..4} (5 alike) : Memory
  Mux{1..4} (4 alike) : Mux  Inputs=3
  "Power (dq0, Instantaneous)" : spsPowerdq0InstantaneousLib/Power (dq0, Instantaneous)
  RL_a : spsSeriesRLCBranchLib/Series RLC Branch  LConnTagsString=__new0  RConnTagsString=__new0  BranchType=RL  Resistance=R_f  Inductance=L_f  SetiL0=off  InitialCurrent=0  Capacitance=1e-6  Setx0=off  InitialVoltage=0  Measurements=Branch voltage and current
  RL_b : spsSeriesRLCBranchLib/Series RLC Branch  LConnTagsString=__new0  RConnTagsString=__new0  BranchType=RL  Resistance=R_f  Inductance=L_f  SetiL0=off  InitialCurrent=0  Capacitance=1e-6  Setx0=off  InitialVoltage=0  Measurements=None
  RL_c : spsSeriesRLCBranchLib/Series RLC Branch  LConnTagsString=__new0  RConnTagsString=__new0  BranchType=RL  Resistance=R_f  Inductance=L_f  SetiL0=off  InitialCurrent=0  Capacitance=1e-6  Setx0=off  InitialVoltage=0  Measurements=None
  Saturation : Saturate  UpperLimit=i_ul  LowerLimit=i_ll
  Sqrt2 : Sqrt
  Sum2 : Sum  Inputs=+++  InputSameDT=on  SaturateOnIntegerOverflow=on
  Switch : Switch  Criteria=u2 > Threshold  Threshold=T_en
  Transfer Fcn2 : TransferFcn  Numerator=[w_f]  Denominator=[1 w_f]
  Universal Bridge : spsUniversalBridgeLib/Universal Bridge  Arms=3  SnubberResistance=1e5  SnubberCapacitance=inf  Device=Average-model based VSC  Ron=1e-3  Lon=0  ForwardVoltages="[  0  0  ]"  ForwardVoltage=0  GTOparameters=[ 10e-6 , 20e-6 ]  IGBTparameters=[ 1e-6 , 2e-6 ]  Measurements=None  Measurements_2=None  converterType=Rectifier
  VSM Control : Subsystem
  Voltage Loop : Subsystem
  Voltage Measurement{,1..6} (7 alike) : spsVoltageMeasurementLib/Voltage Measurement  PhasorSimulation=off  OutputType=Complex  PSBequivalent=0
  abc to dq{1..6} (6 alike) : spsabctodq0Lib/abc to dq0  Alignment=90 degrees behind phase A axis
  dq0 to abc : spsdq0toabcLib/dq0 to abc  Alignment=90 degrees behind phase A axis
  d²2 : Product  InputSameDT=on  RndMeth=Zero  SaturateOnIntegerOverflow=on
  i_dc1 : spsControlledCurrentSourceLib/Controlled Current Source  Initialize=off  Source_Type=DC  Amplitude=i_dc  Phase=0  Frequency=0  Measurements=None
  q²4 : Product  InputSameDT=on  RndMeth=Zero  SaturateOnIntegerOverflow=on
  q²5 : Product  InputSameDT=on  RndMeth=Zero  SaturateOnIntegerOverflow=on
  A : PMIOPort  Side=Right
  B : PMIOPort  Port=2  Side=Right
  C : PMIOPort  Port=3  Side=Right
  f : Outport  VectorParamsAs1DForOutWhenUnconnected=off
  V : Outport  Port=2  VectorParamsAs1DForOutWhenUnconnected=off
  P : Outport  Port=3  VectorParamsAs1DForOutWhenUnconnected=off
  Theta : Outport  Port=4  VectorParamsAs1DForOutWhenUnconnected=off
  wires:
  [v_dc] -> Gain17/1
  [P_s_abc] -> Add2/1
  Add6/1 -> Gain16/1
  [v_dc] -> Add6/2
  Transfer Fcn2/1 -> Gain14/1
  Add2/1 -> Transfer Fcn2/1
  Gain17/1 -> Add4/3
  Constant1/1 -> Add6/1
  Gain16/1 -> Add4/1
  Gain13/1 -> Add4/2
  [P_set] -> Gain13/1
  Gain14/1 -> Add4/4
  [P_abc] -> Add2/2
  Constant4/1 -> VSM Control/3(v_m)
  VSM Control/1(w_ref) -> [w]
  [P_abc] -> VSM Control/1(p_m)
  [v_abc] -> VSM Control/4(V_abc)
  [P_set] -> VSM Control/2(p_set)
  Constant2/1 -> VSM Control/5(w_b)
  VSM Control/3(v_ref_dq0) -> [v_ref_dq0]
  VSM Control/2(theta_ref) -> [theta]
  [v_s_ref_dq0] -> dq0 to abc/1
  Gain19/1 -> Universal Bridge/1
  Switch/1 -> i_dc1/1
  [v_dq0] -> Voltage Loop/2(v_dq0)
  [w] -> Voltage Loop/4(w)
  Current Loop/1(v_s_ref_dq0) -> [v_s_ref_dq0]
  [i_s_dq0] -> Current Loop/3(i_s_dq0)
  [v_dq0] -> Current Loop/2(v_dq0)
  Voltage Loop/1(i_s_ref_dq0) -> Current Loop/1(i_s_ref_dq0)
  [i_dq0] -> Voltage Loop/3(i_dq0)
  [v_ref_dq0] -> Voltage Loop/1(v_ref_dq0)
  [w] -> Current Loop/4(w)
  dq0 to abc/1 -> Gain19/1
  Memory1/1 -> [i_s_abc]
  Memory/1 -> [v_s_abc]
  Memory4/1 -> [v_dc]
  Voltage Measurement/1 -> Memory4/1
  Memory3/1 -> [i_abc]
  Memory2/1 -> [v_abc]
  Mux4/1 -> Memory1/1
  Sqrt2/1 -> [V]
  Demux2/1 -> d²2/2, d²2/1  "d"
  Demux2/2 -> q²4/2, q²4/1  "q"
  d²2/1 -> Sum2/1
  Demux2/3 -> q²5/2, q²5/1  "0"
  Sum2/1 -> Sqrt2/1
  q²5/1 -> Sum2/3
  [v_dq0] -> Demux2/1
  q²4/1 -> Sum2/2
  [theta] -> dq0 to abc/2
  abc to dq6/1 -> [v_dq0]
  abc to dq5/1 -> [v_s_dq0]
  abc to dq4/1 -> [i_s_dq0]
  abc to dq3/1 -> [i_dq0]
  [theta] -> abc to dq3/2, abc to dq6/2, abc to dq5/2, abc to dq4/2
  [v_s_abc] -> abc to dq5/1
  [v_abc] -> abc to dq6/1
  [i_s_abc] -> abc to dq4/1
  [i_abc] -> abc to dq3/1
  [theta] -> Theta/1
  Gain4/1 -> V/1
  [i_abc] -> abc to dq1/1
  "Power (dq0, Instantaneous)"/1 -> [P_abc]
  "Power (dq0, Instantaneous)"/2 -> [Q_abc]
  [v_abc] -> abc to dq2/1
  [theta] -> abc to dq1/2, abc to dq2/2
  abc to dq2/1 -> "Power (dq0, Instantaneous)"/1
  abc to dq1/1 -> "Power (dq0, Instantaneous)"/2
  Mux1/1 -> Memory/1
  Mux3/1 -> Memory3/1
  Mux2/1 -> Memory2/1
  [w] -> Gain12/1
  Gain12/1 -> f/1
  Pset/1 -> Gain2/1
  Gain2/1 -> [P_set]
  [V] -> Gain4/1
  Voltage Measurement1/1 -> Mux1/1
  Voltage Measurement2/1 -> Mux1/2
  Voltage Measurement3/1 -> Mux1/3
  Voltage Measurement6/1 -> Mux2/3
  Voltage Measurement5/1 -> Mux2/2
  Voltage Measurement4/1 -> Mux2/1
  Current Measurement1/1 -> Mux3/1
  Current Measurement2/1 -> Mux3/2
  Current Measurement3/1 -> Mux3/3
  Current Measurement4/1 -> Mux4/1
  Current Measurement5/1 -> Mux4/2
  Current Measurement6/1 -> Mux4/3
  [P_abc] -> Gain7/1
  Gain7/1 -> P/1
  LTI System3/1 -> Saturation/1, Switch/3
  Saturation/1 -> Switch/1
  Clock/1 -> Switch/2
  Add4/1 -> LTI System3/1
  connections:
  RL_c/RConn1 -- C_c1/LConn1 -- Current Measurement1/LConn1 -- Voltage Measurement4/LConn1
  C_c1/RConn1 -- Ground2/LConn1 -- C_a/RConn1 -- C_b/RConn1
  i_dc1/LConn1 -- G_dc1/RConn1 -- C_dc1/RConn1 -- Voltage Measurement/LConn2 -- Universal Bridge/RConn2
  Voltage Measurement1/LConn1 -- Current Measurement4/LConn1 -- Universal Bridge/LConn1
  Voltage Measurement2/LConn1 -- Current Measurement5/LConn1 -- Universal Bridge/LConn2
  Voltage Measurement3/LConn1 -- Universal Bridge/LConn3 -- Current Measurement6/LConn1
  Current Measurement1/RConn1 -- A/RConn1
  Current Measurement2/RConn1 -- B/RConn1
  Current Measurement3/RConn1 -- C/RConn1
  Voltage Measurement3/LConn2 -- Voltage Measurement1/LConn2 -- Voltage Measurement2/LConn2 -- Ground/LConn1
  Ground1/LConn1 -- Voltage Measurement4/LConn2 -- Voltage Measurement5/LConn2 -- Voltage Measurement6/LConn2
  i_dc1/RConn1 -- G_dc1/LConn1 -- C_dc1/LConn1 -- Universal Bridge/RConn1 -- Voltage Measurement/LConn1
  Current Measurement5/RConn1 -- RL_b/LConn1
  Current Measurement6/RConn1 -- RL_a/LConn1
  Current Measurement4/RConn1 -- RL_c/LConn1
  RL_a/RConn1 -- C_a/LConn1 -- Current Measurement3/LConn1 -- Voltage Measurement6/LConn1
  C_b/LConn1 -- Current Measurement2/LConn1 -- Voltage Measurement5/LConn1 -- RL_b/RConn1
